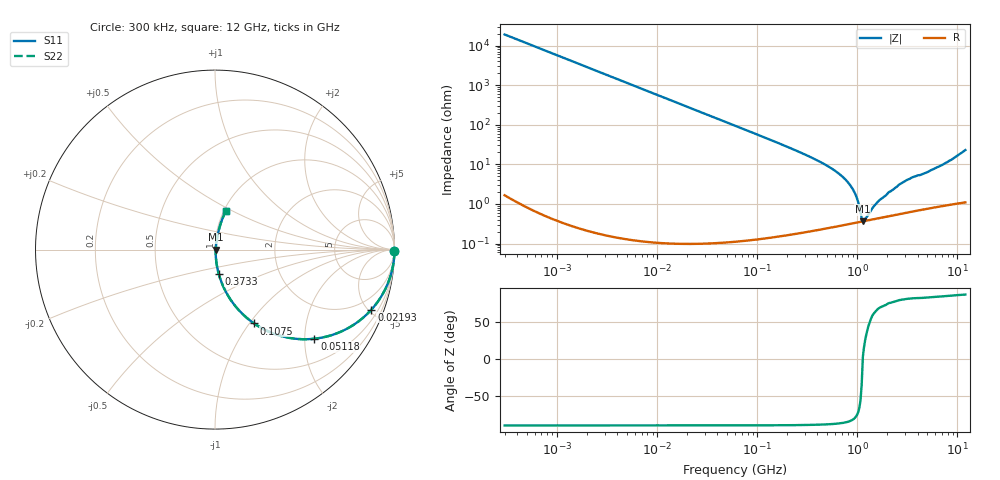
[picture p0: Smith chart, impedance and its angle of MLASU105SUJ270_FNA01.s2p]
! MLASU105SUJ270_FNA01  S-PARAMETER MODEL  ( General Type )
! Model Generated by TAIYO YUDEN Corporation (http://www.ty-top.com)
! Version 3.0
! TAIYO YUDEN Control No. 120810
! Copyright(c) 2003 TAIYO YUDEN CO.,LTD. All Rights Reserved.
! Product Description (link to TY-COMPAS)
! https://ds.yuden.co.jp/TYCOMPAS/or/detail?pn=MLASU105SUJ270JFNA01&u=M
! Products Name : Multilayer Ceramic Capacitors
! Characteristics :
!  Capacitance : 27 pF , Rated Voltage : 50V , TCC : UJ / U2J
!  Case Size : 1.0 x 0.5 / 0.039 x 0.02 [mm/inch] , Thickness : 0.5 / 0.02 [mm/inch]
!  (Conditions: Temperature = 25 degC , DC Bias Current/Voltage = 0A / 0V)
! External Node Assignments :
!  1  o---| |---o  2
! GND o---------o GND
! Frequency Range : 0.3MHz  -  12000MHz  [ 401 STEP ]
# MHz S RI R 50
! Freq[MHz].  S11 Real  S11 Imag  S21 Real  S21 Imag  S12 Real  S12 Imag  S22 Real  S22 Imag
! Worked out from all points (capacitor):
!   401 points, 300 kHz to 12 GHz, reference 50 ohm
!   read as one part in series: C = 27.9 pF near 316.3 kHz
!   lowest |Z| = 363 mohm at 1.136 GHz (marker M1)
!   series resonance near 1.133 GHz, so ESL is about 710 pH
!   S11 on the Smith chart (normalised r, x): 300 kHz: open; 21.93 MHz: 1.00, -5.21; 51.18 MHz: 1.00, -2.23; 107.5 MHz: 1.00, -1.05; 373.3 MHz: 1.00, -0.27; 12 GHz: 1.02, +0.46
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0.3  1 -0.00525  2.81e-05 0.00525  2.81e-05 0.00525  1 -0.00525
1.769972  0.999 -0.031  0.000962 0.031  0.000962 0.031  0.999 -0.031
10.44266  0.9676 -0.177  0.0324 0.177  0.0324 0.177  0.9676 -0.177
21.92581  0.8713 -0.3347  0.1287 0.3347  0.1287 0.3347  0.8713 -0.3347
51.18236  0.5534 -0.4967  0.4466 0.4967  0.4466 0.4967  0.5534 -0.4967
60  0.4739 -0.4987  0.5261 0.4987  0.5261 0.4987  0.4739 -0.4987
107.4644  0.2177 -0.4114  0.7823 0.4114  0.7823 0.4114  0.2177 -0.4114
182.544  0.0861 -0.278  0.9139 0.278  0.9139 0.278  0.0861 -0.278
353.9943  0.0227 -0.142  0.9773 0.142  0.9773 0.142  0.0227 -0.142
373.2558  0.0203 -0.1333  0.9797 0.1333  0.9797 0.1333  0.0203 -0.1333
601.3112  0.00723 -0.0675  0.9928 0.0675  0.9928 0.0675  0.00723 -0.0675
804.7407  0.00427 -0.0349  0.9957 0.0349  0.9957 0.0349  0.00427 -0.0349
894.6982  0.00378 -0.0238  0.9962 0.0238  0.9962 0.0238  0.00378 -0.0238
968.706  0.00359 -0.0157  0.9964 0.0157  0.9964 0.0157  0.00359 -0.0157
1076.992  0.00354 -0.00506  0.9965 0.00506  0.9965 0.00506  0.00354 -0.00506
1135.593  0.00361 0.000194  0.9964 -0.000194  0.9964 -0.000194  0.00361 0.000194
1197.383  0.00371 0.00179  0.9963 -0.00179  0.9963 -0.00179  0.00371 0.00179
1519.776  0.00426 0.00871  0.9957 -0.00871  0.9957 -0.00871  0.00426 0.00871
2088.533  0.00529 0.0194  0.9947 -0.0194  0.9947 -0.0194  0.00529 0.0194
3026.31  0.0073 0.0373  0.9927 -0.0373  0.9927 -0.0373  0.0073 0.0373
6699.894  0.0164 0.0881  0.9836 -0.0881  0.9836 -0.0881  0.0164 0.0881
12000  0.0594 0.2137  0.9406 -0.2137  0.9406 -0.2137  0.0594 0.2137
